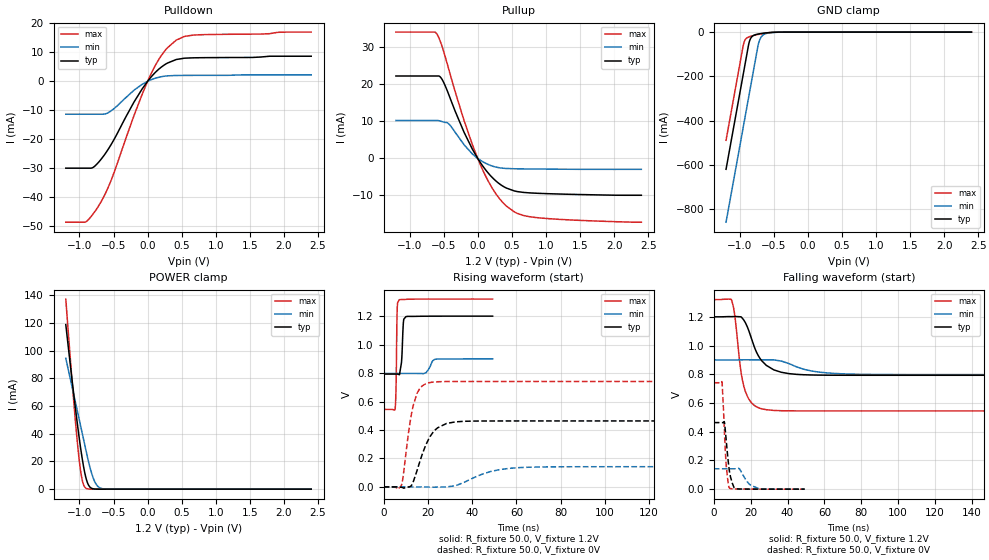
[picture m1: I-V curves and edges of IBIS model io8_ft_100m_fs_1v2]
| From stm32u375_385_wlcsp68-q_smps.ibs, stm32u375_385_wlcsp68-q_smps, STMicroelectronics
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[Model]   io8_ft_100m_fs_1v2
Model_type I/O
Polarity   Non-Inverting
Enable   Active-Low
| CAP_THRESHOLD on pad IOFT is "UDTCAPC" :
| Rising=30.0% of vddiom   Falling=70.0% of vddiom
| C_comp min and max val. don't necessarily correlate with the min and max pvt
| but are the smallest and greatest pad capacitance found.
| var   typ   min   max
C_comp   2.92097pF  2.86112pF  2.97372pF
|C_comp_pullup   1.65811pF  1.48846pF  1.79608pF
|C_comp_pulldown   1.26287pF  1.37266pF  1.17763pF
Vinl = 450.0mV
Vinh = 660.0mV
Vmeas = 600.0mV   | Reference voltage for timing measurements
Cref  = 50.0pF   | Timing specification test load capacitance value
Rref  = 1.0MOhm   | Timing specification test load resistance value
Vref  = 660.0mV   | Timing specification test load voltage
[Model Spec]
| TIME_THRESHOLD on pin ZIV11 is "CMOS" :
| Rising=50.0% of vdd   Falling=50.0% of vdd
Vinl 439.50000mV 331.50001mV 485.50000mV
Vinh 752.50000mV 552.50001mV 837.50000mV
| variable   typ   min   max
[Temperature Range] 25.0 130.0 -40.0
| variable   typ   min   max
[Voltage Range] 1.2V 900.0mV 1.32V
| variable   typ   min   max
[POWER Clamp Reference] 1.2V 900.0mV 1.32V
| variable   typ   min   max
[GND Clamp Reference] 0V 0V 0V
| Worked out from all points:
|   slope of the pulldown table from 0 to 0.18 V, typ, clamps not added: 40 ohm
|   slope of the pullup table from 0 to 0.18 V, typ, clamps not added: 40 ohm
|   GND clamp passes 1 mA (typ) near -0.50 V on its own axis
|   POWER clamp passes 1 mA (typ) near -0.83 V on its own axis
|   rising waveform, R_fixture 50.0, V_fixture 1.2V: 20-80 % time 717ps typ, 1.98ns min, 395ps max; typ from 0.793 V to 1.2 V
|   falling waveform, R_fixture 50.0, V_fixture 1.2V: 20-80 % time 8.98ns typ, 16ns min, 4.87ns max; typ from 1.2 V to 0.793 V
|   rising waveform, R_fixture 50.0, V_fixture 0V: 20-80 % time 7.11ns typ, 14.2ns min, 4.39ns max; typ from 0 V to 0.464 V
|   falling waveform, R_fixture 50.0, V_fixture 0V: 20-80 % time 2.43ns typ, 4.78ns min, 1.78ns max; typ from 0.464 V to 0 V
[POWER Clamp]
-1.2V     118.8mA    94.44mA    137.2mA
-1.09V    71.2mA     69.75mA    67.14mA
-1.02V    43.22mA    54.03mA    28.67mA
-990mV    32.26mA    47.3mA     15.78mA
-970mV    25.49mA    42.81mA    9.257mA
-940mV    16.45mA    36.08mA    3.257mA
-910mV    9.238mA    29.34mA    904.6uA
-860mV    2.387mA    18.53mA    87.46uA
-790mV    204.6uA    7.049mA    3.101uA
-730mV    21.91uA    2.041mA    176.4nA
-660mV    1.594uA    337.6uA    6.285nA
2.4V      0A         0A         0A
[GND Clamp]
-1.2V     -619mA     -857.5mA   -488.2mA
-950mV    -194mA     -432.5mA   -63.18mA
-930mV    -160mA     -398.5mA   -40.87mA
-870mV    -57.95mA   -296.5mA   -22.39mA
-840mV    -28.97mA   -245.5mA   -19.16mA
-800mV    -15.67mA   -177.5mA   -15.71mA
-730mV    -8.807mA   -59.89mA   -10.55mA
-700mV    -7.204mA   -30.66mA   -8.61mA
-660mV    -5.427mA   -13.83mA   -6.309mA
-580mV    -2.713mA   -4.125mA   -2.796mA
-380mV    -62.64uA   -240.2uA   -21.17uA
2.4V      836.4pA    121.5nA    348.6pA
| variable   typ   min   max
[Pullup Reference] 1.2V 900.0mV 1.32V
| variable   typ   min   max
[Pulldown Reference] 0V 0V 0V
[Pullup]
-1.2V     22.27mA    10.26mA    34.13mA
-630mV    22.27mA    10.26mA    34.13mA
-600mV    22.27mA    10.26mA    33.65mA
-530mV    21.55mA    10mA       30.63mA
-420mV    17.01mA    9.25mA     23.77mA
-200mV    7.047mA    3.686mA    10.21mA
-10mV     299.4uA    135.1uA    455.2uA
200mV     -4.898mA   -1.964mA   -7.619mA
420mV     -8mA       -2.709mA   -12.87mA
580mV     -8.947mA   -2.8mA     -14.83mA
790mV     -9.331mA   -2.845mA   -15.82mA
2.4V      -9.943mA   -2.948mA   -17.22mA
[Pulldown]
-1.2V     -29.93mA   -11.33mA   -48.55mA
-910mV    -29.93mA   -11.33mA   -48.48mA
-810mV    -29.8mA    -11.33mA   -46.03mA
-710mV    -27.65mA   -11.33mA   -42.6mA
-620mV    -24.89mA   -11.22mA   -38.69mA
-530mV    -21.58mA   -10.08mA   -33.79mA
-200mV    -7.157mA   -3.075mA   -11.82mA
40mV      1.18mA     424.7uA    2.081mA
230mV     5.395mA    1.701mA    9.799mA
420mV     7.512mA    2.016mA    14.19mA
670mV     8.097mA    2.046mA    15.93mA
2.4V      8.645mA    2.222mA    16.96mA
[Ramp]
dV/dt_r 278.1365mV/7.08165ns 85.18305mV/13.92889ns 444.65369mV/4.28926ns
dV/dt_f 244.21065mV/8.84393ns 61.56309mV/15.62989ns 465.10837mV/4.83875ns
R_load = 50.0
| Removed startup time: 0s 0s 0s  .
| Removed end time: 49.25ns.
[Rising Waveform]
R_fixture   = 50.0
V_fixture   = 1.2V
V_fixture_min = 900.0mV
V_fixture_max = 1.32V
0s        793mV      797.4mV    544.8mV
5.2ns     793mV      797.4mV    551.6mV
5.6ns     793.1mV    797.4mV    698.7mV
6.15ns    792.9mV    797.4mV    1.259V
7.05ns    788.9mV    797.4mV    1.315V
8.05ns    872.9mV    797.4mV    1.317V
9ns       1.168V     797.4mV    1.317V
10.05ns   1.197V     797.4mV    1.318V
23.15ns   1.2V       896.6mV    1.32V
49.25ns   1.2V       899.9mV    1.32V
| Removed startup time: 0s 0s 0s  .
| Removed end time: 199.25ns.
[Falling Waveform]
R_fixture   = 50.0
V_fixture   = 1.2V
V_fixture_min = 900.0mV
V_fixture_max = 1.32V
0s        1.2V       900mV      1.32V
9.65ns    1.201V     900mV      1.317V
11.25ns   1.202V     900mV      1.222V
14.25ns   1.2V       900.5mV    865.6mV
16.25ns   1.178V     900.6mV    718.4mV
20.35ns   1.052V     900.5mV    602.4mV
25.2ns    907.7mV    900.5mV    562.6mV
32.55ns   830.6mV    900.1mV    548.2mV
48.8ns    796.6mV    834.8mV    544.9mV
199.3ns   793mV      797.4mV    544.8mV
| Removed startup time: 0s 0s 0s  .
| Removed end time: 199.2ns.
[Rising Waveform]
R_fixture   = 50.0
V_fixture   = 0V
V_fixture_min = 0V
V_fixture_max = 0V
0s        4.598nV    136nV      3.245nV
8ns       -2.564mV   877.9nV    10.08mV
11.65ns   527.5uV    182.7nV    424.8mV
13.3ns    32.33mV    -624.3nV   567.6mV
16.25ns   173.4mV    40.42uV    690.2mV
20.35ns   336.3mV    -980.9uV   731.5mV
24.4ns    415.4mV    -890.8uV   739mV
36.6ns    461.2mV    33.75mV    741mV
61ns      463.4mV    135.4mV    741mV
199.2ns   463.6mV    142mV      741.1mV
| Removed startup time: 0s 0s 0s  .
| Removed end time: 49.25ns.
[Falling Waveform]
R_fixture   = 50.0
V_fixture   = 0V
V_fixture_min = 0V
V_fixture_max = 0V
0s        463.6mV    142mV      741.1mV
4.45ns    463.6mV    142mV      746.3mV
5.7ns     469.6mV    142mV      423.6mV
6.6ns     360.1mV    142mV      192.2mV
7.8ns     198.2mV    142mV      44.02mV
8.55ns    119.2mV    142mV      6.737mV
10.05ns   41.43mV    142mV      2.233mV
12.05ns   2.293mV    141.8mV    1.013mV
24.15ns   229uV      6.317mV    43.43uV
49.25ns   5.643uV    116.2uV    18.18nV
